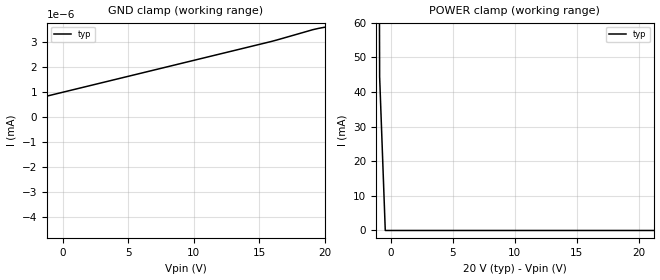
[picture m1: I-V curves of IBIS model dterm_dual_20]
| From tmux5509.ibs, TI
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| dterm_dual_20
[Model]   dterm_dual_20
Model_type   Terminator
|   typ   min   max
C_comp   6.362683e-12   NA   NA
[Voltage Range]   20   NA   NA
[Temperature Range]   27   NA   NA
[Power Clamp Reference]   20   NA   NA
[GND Clamp Reference]   0   NA   NA
[GND Clamp]
|   Voltage   I(typ)   I(min)   I(max)
-25V      -2.839A    NA         NA
-20.45V   -1.081uA   NA         NA
-20V      -1.588nA   NA         NA
-15.91V   -1.034nA   NA         NA
15.91V    3.008nA    NA         NA
19.09V    3.479nA    NA         NA
20V       3.577nA    NA         NA
[POWER Clamp]
|   Voltage   I(typ)   I(min)   I(max)
-5V       7.432A     NA         NA
-1.364V   581.6mA    NA         NA
-909.1mV  44.4mA     NA         NA
-454.5mV  510.4nA    NA         NA
40V       -3.008nA   NA         NA
